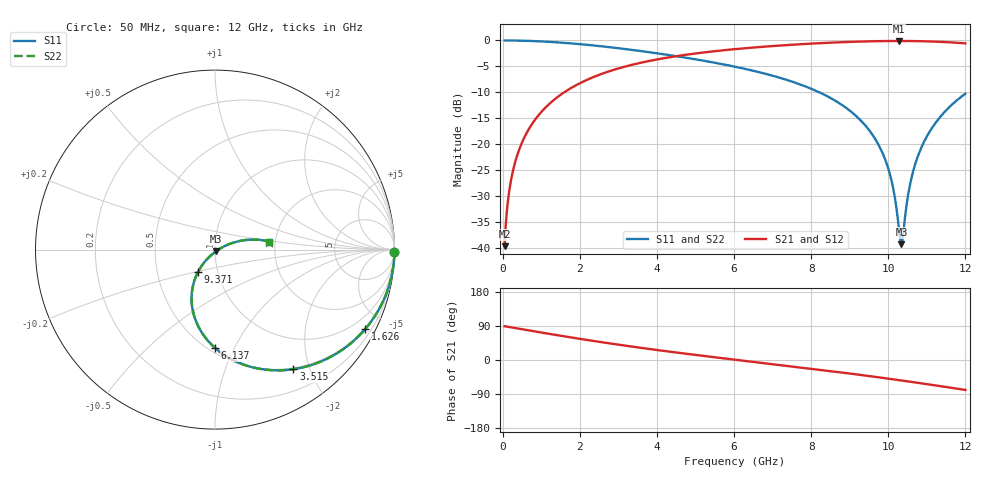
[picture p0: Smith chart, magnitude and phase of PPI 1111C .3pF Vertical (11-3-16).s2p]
# GHz S MA R 50
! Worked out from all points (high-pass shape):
!   1601 points, 50 MHz to 12 GHz, reference 50 ohm
!   highest |S21| = -0.10 dB at 10.27 GHz (marker M1); lowest = -39.7 dB at 50 MHz (marker M2)
!   |S21| within 3 dB of the highest: 4.444 GHz to end of sweep
!   lowest |S11| = -39.3 dB at 10.34 GHz (marker M3), VSWR 1.02, Z = 50.7 - j0.861 ohm
!   |S11| at or under -10 dB: 8.211 GHz to end of sweep
!   |S22| runs from -39.3 to 0.0 dB; largest |S21 - S12| = 0
!   S11 on the Smith chart (normalised r, x): 50 MHz: open; 1.626 GHz: 0.46, -3.96; 3.515 GHz: 0.48, -1.75; 6.137 GHz: 0.54, -0.84; 9.371 GHz: 0.80, -0.21; 12 GHz: 1.86, +0.18
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0.05  0.9999 -0.9  0.0104 89.1  0.0104 89.1  0.9999 -0.9
0.1470937  0.9995 -2.6  0.03058 87.4  0.03058 87.4  0.9995 -2.6
0.2217813  0.9989 -3.9  0.04608 86.1  0.04608 86.1  0.9989 -3.9
0.4906563  0.9948 -8.6  0.1016 81.4  0.1016 81.4  0.9948 -8.6
0.94625  0.981 -16.5  0.1934 73.4  0.1934 73.4  0.981 -16.5
1.625906  0.9464 -28.0  0.3218 62.0  0.3218 62.0  0.9464 -28.0
2.044156  0.9185 -34.8  0.394 55.1  0.394 55.1  0.9185 -34.8
3.5155  0.7965 -56.8  0.602 33.1  0.602 33.1  0.7965 -56.8
4.038312  0.7486 -63.9  0.6599 25.9  0.6599 25.9  0.7486 -63.9
6.025  0.5582 -88.7  0.8247 0.8  0.8247 0.8  0.5582 -88.7
6.137031  0.547 -90.1  0.832 -0.6  0.832 -0.6  0.547 -90.1
8.019156  0.3401 -112.1  0.9329 -23.3  0.9329 -23.3  0.3401 -112.1
9.371  0.1567 -127.2  0.9781 -40.6  0.9781 -40.6  0.1567 -127.2
9.744438  0.09913 -130.0  0.9849 -45.6  0.9849 -45.6  0.09913 -130.0
10.01331  0.05599 -128.8  0.9877 -49.4  0.9877 -49.4  0.05599 -128.8
10.15522  0.03309 -122.9  0.9885 -51.4  0.9885 -51.4  0.03309 -122.9
10.27472  0.01542 -99.1  0.9887 -53.1  0.9887 -53.1  0.01542 -99.1
10.34194  0.01082 -51.7  0.9887 -54.0  0.9887 -54.0  0.01082 -51.7
10.58841  0.04498 17.9  0.9873 -57.6  0.9873 -57.6  0.04498 17.9
10.86475  0.09398 21.2  0.9833 -61.7  0.9833 -61.7  0.09398 21.2
11.33528  0.1809 17.3  0.9704 -68.7  0.9704 -68.7  0.1809 17.3
12  0.3069 8.4  0.9375 -79.0  0.9375 -79.0  0.3069 8.4
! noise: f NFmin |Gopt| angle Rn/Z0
0.05  0.002615  0.9897  0.8699  0.05791
1.372  0.005994  0.8133  12.87  0.00662
2.701  0.009377  0.7522  19.64  0.007417
4.031  0.01258  0.7247  26.1  0.008626
5.36  0.01578  0.7124  32.4  0.009998
6.682  0.01906  0.7098  38.46  0.01156
8.012  0.02259  0.7142  44.32  0.01344
9.341  0.02648  0.7242  49.93  0.01575
10.67  0.03089  0.7388  55.29  0.01869
12  0.03602  0.7572  60.42  0.02256
